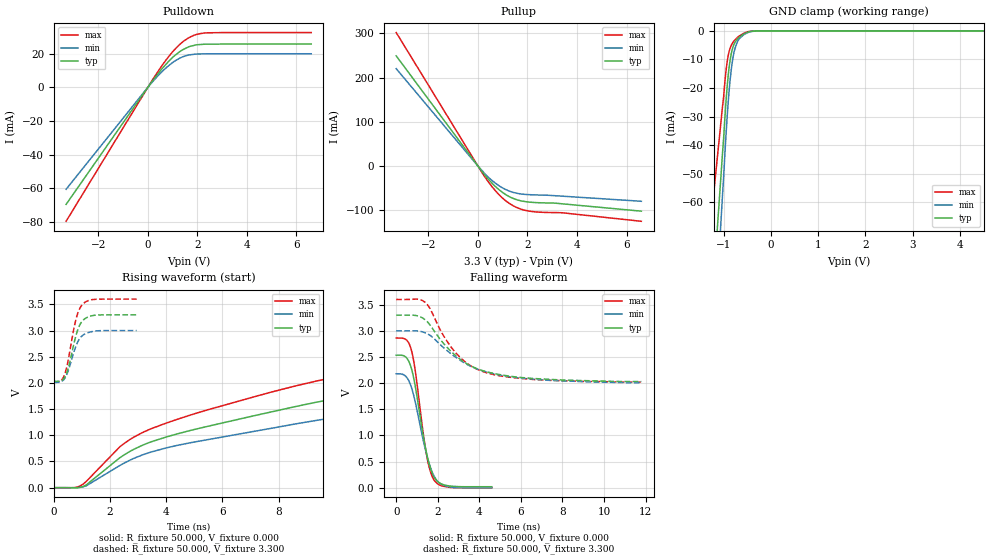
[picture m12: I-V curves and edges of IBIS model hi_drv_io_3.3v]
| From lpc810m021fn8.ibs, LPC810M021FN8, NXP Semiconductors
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[Model]   hi_drv_io_3.3v
Model_type I/O
Vinl=9.900E-01
Vinh=2.310E+00
Vref=0.000E+00
Rref=1.000E+06
Cref=2.000E-11
Vmeas=1.650E+00
C_comp   8.440E-13   8.280E-13   8.600E-13
[Voltage Range]   3.300E+00   3.000E+00   3.600E+00
[POWER Clamp Reference]   3.300E+00   3.000E+00   3.600E+00
[GND Clamp Reference]   0.000E+00   0.000E+00   0.000E+00
[Pullup Reference]   3.300E+00   3.000E+00   3.600E+00
[Pulldown Reference]   0.000E+00   0.000E+00   0.000E+00
[Temperature Range]   25   85   -40
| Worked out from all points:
|   slope of the pulldown table from 0 to 0.495 V, typ, clamps not added: 51.2 ohm
|   slope of the pullup table from 0 to 0.495 V, typ, clamps not added: 14.4 ohm
|   GND clamp passes 1 mA (typ) near -0.56 V on its own axis
|   rising waveform, R_fixture 50.000, V_fixture 0.000: 20-80 % time 11.4ns typ, 13.1ns min, 9.86ns max; typ from 0 V to 2.52 V
|   falling waveform, R_fixture 50.000, V_fixture 0.000: 20-80 % time 666ps typ, 753ps min, 591ps max; typ from 2.53 V to 0.018 V
|   rising waveform, R_fixture 50.000, V_fixture 3.300: 20-80 % time 360ps typ, 375ps min, 352ps max; typ from 2.03 V to 3.3 V
|   falling waveform, R_fixture 50.000, V_fixture 3.300: 20-80 % time 2.09ns typ, 2.46ns min, 1.77ns max; typ from 3.3 V to 2.03 V
[GND Clamp]
-3.3V     -590.4mA   -698mA     -398.8mA
-1.02V    -42.46mA   -57.07mA   -26.24mA
-1V       -38.06mA   -51.76mA   -23.49mA
-960mV    -27.61mA   -39.88mA   -15.89mA
-920mV    -18.88mA   -29.31mA   -10.45mA
-880mV    -12.49mA   -20.65mA   -7.085mA
-820mV    -6.778mA   -11.45mA   -4.527mA
-780mV    -4.748mA   -7.624mA   -3.589mA
-720mV    -3.081mA   -4.344mA   -2.525mA
-560mV    -993.4uA   -1.241mA   -739uA
-280mV    0A         0A         0A
6.6V      0A         0A         0A
[POWER Clamp]
-3.3V     0A         0A         0A
6.6V      0A         0A         0A
[Pullup]
-3.3V     249.2mA    220.2mA    301.9mA
200mV     -14.86mA   -12.4mA    -18.13mA
440mV     -31.15mA   -26.44mA   -37.26mA
700mV     -46.18mA   -38.59mA   -55.7mA
1.12V     -64.6mA    -53.15mA   -78.67mA
1.56V     -76.12mA   -61.5mA    -93.77mA
2.1V      -81.83mA   -64.95mA   -102.3mA
3.44V     -85.76mA   -68.42mA   -106.1mA
6.6V      -102.2mA   -79.85mA   -125.1mA
[Pulldown]
-3.3V     -69.61mA   -60.63mA   -79.67mA
160mV     3.297mA    2.832mA    3.818mA
600mV     11.55mA    9.76mA     13.55mA
900mV     16.39mA    13.61mA    19.41mA
1.08V     18.87mA    15.6mA     22.43mA
1.44V     22.62mA    18.34mA    27.44mA
1.86V     24.96mA    19.68mA    30.98mA
2.4V      25.7mA     20mA       32.46mA
6.6V      25.77mA    20.01mA    32.62mA
[Rising Waveform]
R_fixture = 50.000
V_fixture = 0.000
V_fixture_min = 0.000
V_fixture_max = 0.000
|  time   V(typ)   V(min)   V(max)
0s        0V         0V         0V
950ps     7.514mV    7.644mV    36.36mV
2.5ns     625.3mV    468.2mV    842.9mV
4ns       967.3mV    759mV      1.233V
8.65ns    1.554V     1.222V     1.949V
12.8ns    1.952V     1.566V     2.382V
16.05ns   2.171V     1.774V     2.586V
20.75ns   2.344V     1.972V     2.726V
26.35ns   2.439V     2.089V     2.805V
35.65ns   2.517V     2.179V     2.872V
[Falling Waveform]
R_fixture = 50.000
V_fixture = 0.000
V_fixture_min = 0.000
V_fixture_max = 0.000
|  time   V(typ)   V(min)   V(max)
0s        2.534V     2.179V     2.864V
450ps     2.502V     2.134V     2.839V
750ps     2.255V     1.896V     2.602V
950ps     1.864V     1.579V     2.143V
1.45ns    679.9mV    657.1mV    650.5mV
1.6ns     429.9mV    445.8mV    369.9mV
1.8ns     217.3mV    239mV      160.6mV
2.1ns     86.74mV    84.24mV    49.28mV
2.5ns     37.05mV    20.25mV    10.53mV
4.6ns     17.89mV    0V         -3.688mV
[Rising Waveform]
R_fixture = 50.000
V_fixture = 3.300
V_fixture_min = 3.000
V_fixture_max = 3.600
|  time   V(typ)   V(min)   V(max)
0s        2.03V      2.009V     2.019V
250ps     2.041V     2.023V     2.044V
400ps     2.118V     2.096V     2.184V
550ps     2.355V     2.293V     2.545V
700ps     2.714V     2.565V     3V
800ps     2.928V     2.721V     3.24V
900ps     3.081V     2.831V     3.397V
1.05ns    3.202V     2.918V     3.515V
1.5ns     3.294V     2.992V     3.597V
2.95ns    3.3V       3V         3.6V
[Falling Waveform]
R_fixture = 50.000
V_fixture = 3.300
V_fixture_min = 3.000
V_fixture_max = 3.600
|  time   V(typ)   V(min)   V(max)
0s        3.3V       3V         3.6V
950ps     3.293V     2.999V     3.607V
1.4ns     3.21V      2.962V     3.542V
1.65ns    3.1V       2.908V     3.409V
2.25ns    2.772V     2.689V     2.925V
2.8ns     2.546V     2.513V     2.61V
3.45ns    2.36V      2.349V     2.367V
4.2ns     2.232V     2.229V     2.217V
6.75ns    2.085V     2.072V     2.066V
11.8ns    2.03V      2.009V     2.019V
[Ramp]
dV/dt_r   1.5096E+00/1.1408E-08   1.3070E+00/1.3103E-08   1.7205E+00/9.8768E-09
dV/dt_f   7.6204E-01/2.0907E-09   5.9483E-01/2.4504E-09   9.4867E-01/1.7686E-09
R_load = 50
